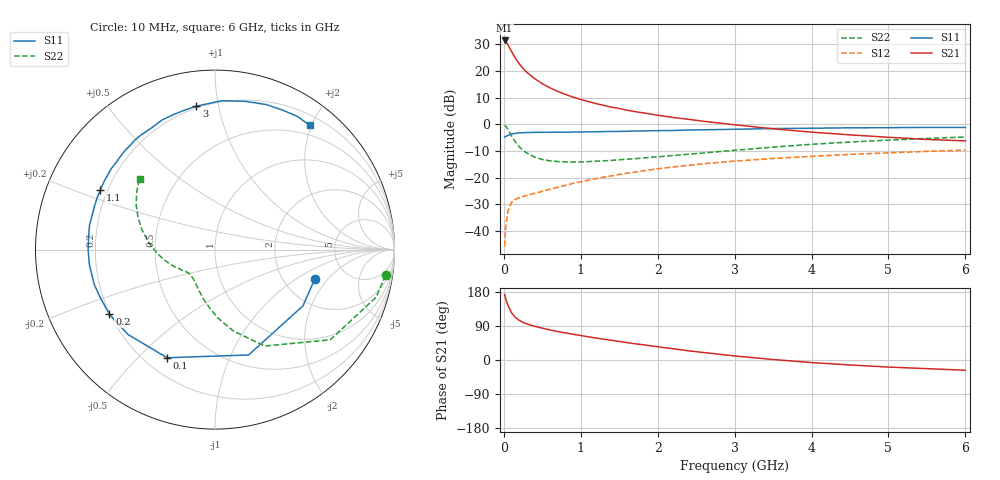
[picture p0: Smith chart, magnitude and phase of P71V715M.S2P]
! SIEMENS Small Signal Semiconductors
! BFP196
! Si NPN RF Bipolar Junction Transistor in SOT143
! VCE = 1.75 V  IC = 15 mA
! Common Emitter S-Parameters:  May  1996
# GHz  S  MA  R  50
!  f  S11  S21  S12  S22
! GHz  MAG  ANG  MAG  ANG  MAG  ANG  MAG  ANG
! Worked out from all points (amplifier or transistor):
!   36 points, 10 MHz to 6 GHz, reference 50 ohm
!   highest |S21| = 31.4 dB at 10 MHz (marker M1)
!   |S21| within 3 dB of that: start of sweep to 79.12 MHz
!   unconditionally stable (mu >= 1): 737.2 MHz to 3.453 GHz
!   at 250 MHz: K = 0.52, MSG = 24.0 dB, |S12| = -27.1 dB
!   at 1.4 GHz: K = 1.13, MAG = 10.7 dB, |S12| = -19.3 dB
!   at 6 GHz: K = 0.99, MSG = 1.7 dB, |S12| = -9.7 dB
!   S11 on the Smith chart (normalised r, x): 10 MHz: 2.94, -1.47; 100 MHz: 0.29, -0.61; 200 MHz: 0.20, -0.27; 1.1 GHz: 0.17, +0.24; 3 GHz: 0.19, +0.86; 6 GHz: 0.34, +1.97
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0.01  0.5793 -16.7  37.15 173.1  0.0052 84.2  0.9609 -8.6
0.02  0.5818 -32.6  35.97 164.7  0.0103 77.5  0.9357 -16.5
0.05  0.6162 -72.3  31.5 145.7  0.0229 61.2  0.8157 -38.0
0.1  0.6589 -113.9  23.11 124.7  0.0344 45.8  0.6048 -62.7
0.15  0.6774 -135.7  17.24 112.4  0.0393 39.5  0.4647 -77.3
0.2  0.6894 -148.6  13.63 104.6  0.0421 37.1  0.3793 -87.9
0.25  0.693 -157.3  11.07 99.1  0.0444 36.6  0.3223 -95.9
0.3  0.7005 -164.0  9.377 95.1  0.0466 37.4  0.2881 -102.0
0.4  0.7054 -173.6  7.161 89.0  0.051 39.4  0.2424 -112.1
0.5  0.7069 -180.0  5.74 84.0  0.0552 41.3  0.2184 -119.3
0.6  0.7081 174.0  4.806 79.3  0.0606 43.4  0.2065 -124.6
0.7  0.7123 168.9  4.138 75.0  0.0659 45.3  0.2002 -129.1
0.9  0.7137 160.4  3.227 67.9  0.0779 47.6  0.1957 -135.9
1.1  0.7202 152.4  2.657 61.2  0.0895 48.5  0.2001 -140.6
1.3  0.7287 144.9  2.255 54.9  0.1025 48.4  0.2061 -144.6
1.6  0.7396 135.5  1.834 45.9  0.1207 47.5  0.2217 -150.1
2.2  0.7642 117.8  1.34 29.7  0.1585 42.7  0.2591 -160.8
3  0.8059 97.4  0.977 10.7  0.2042 33.9  0.3255 -176.9
3.5  0.8303 87.4  0.823 1.3  0.2284 27.9  0.3724 173.6
4.5  0.8571 70.6  0.632 -13.2  0.2724 16.7  0.4646 157.3
5.5  0.8727 58.3  0.519 -22.8  0.3108 5.8  0.5427 143.5
6  0.8711 52.7  0.488 -27.0  0.328 -0.2  0.5766 136.8
